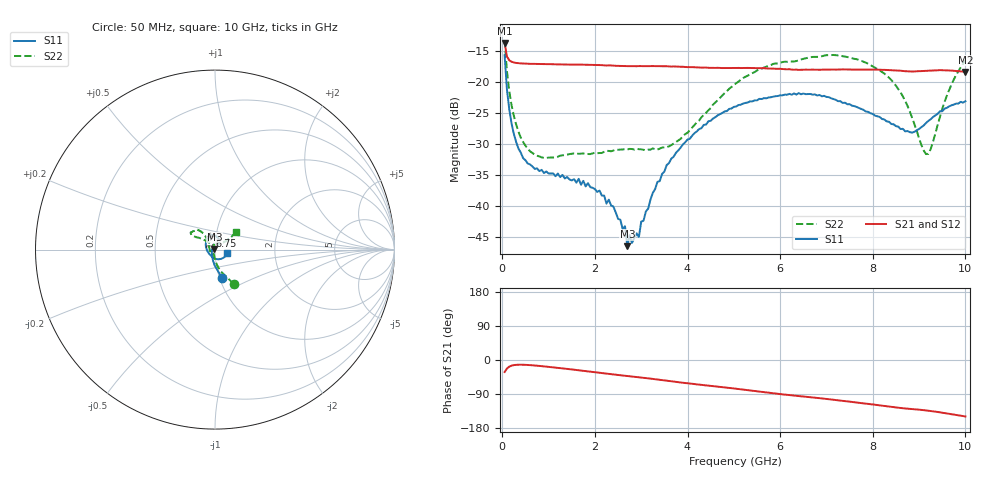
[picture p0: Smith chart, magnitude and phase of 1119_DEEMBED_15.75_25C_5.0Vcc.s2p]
!Hittite Microwave Corp.
!Digital Attenuator/PhaseShifter Rev 1.4.0
!Filename: C:\DATA\DATA\1119_DEEMBED_15.75_25C_5.0Vcc.s2p
!VNA ID: Agilent Technologies,N5224A,MY51441122,A.10.45.03
!Device type:
!2 Port Calibration.
!Temp(C): 25
!Lot Number:
!Serial Number:
!Operator:
!Misc:
!Attenuator:  15.750
# GHZ S DB R 50.0
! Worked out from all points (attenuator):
!   200 points, 50 MHz to 10 GHz, reference 50 ohm
!   highest |S21| = -13.64 dB at 50 MHz (marker M1); lowest = -18.3 dB at 10 GHz (marker M2)
!   lowest |S11| = -46.4 dB at 2.7 GHz (marker M3), VSWR 1.01, Z = 49.7 + j0.382 ohm
!   |S11| at or under -10 dB: start of sweep to end of sweep
!   |S22| runs from -32.2 to -13.2 dB; largest |S21 - S12| = 0.00047
!   S11 on the Smith chart (normalised r, x): 50 MHz: 1.03, -0.34; 6.75 GHz: 0.94, +0.14; 10 GHz: 1.14, -0.05
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0.05  -15.62 -75.7  -13.64 -31.8  -13.64 -31.8  -13.25 -61.3
0.1  -21.12 -91.5  -15.82 -22.7  -15.82 -22.7  -18.18 -75.9
0.2  -26.64 -108.2  -16.68 -14.9  -16.69 -14.9  -23.70 -87.3
0.5  -32.57 -138.9  -16.99 -12.8  -16.99 -12.7  -30.21 -99.6
0.85  -34.12 -159.5  -17.05 -16.2  -17.05 -16.2  -32.12 -106.4
1.75  -35.90 -178.8  -17.16 -28.6  -17.16 -28.6  -31.47 -116.7
2.3  -38.93 165.0  -17.27 -36.6  -17.27 -36.7  -31.07 -132.0
2.65  -43.22 131.8  -17.38 -41.6  -17.39 -41.6  -30.77 -141.7
2.7  -46.43 126.5  -17.38 -42.2  -17.39 -42.3  -30.84 -142.6
2.75  -44.64 119.1  -17.40 -42.9  -17.40 -43.0  -30.74 -144.7
2.95  -44.93 89.4  -17.38 -45.5  -17.39 -45.6  -30.79 -153.9
3.4  -35.94 62.6  -17.40 -52.2  -17.41 -52.3  -30.70 -176.9
4  -29.24 58.0  -17.55 -61.4  -17.56 -61.4  -28.14 149.1
5.05  -23.90 70.6  -17.69 -75.8  -17.71 -75.9  -20.15 125.3
6.7  -21.99 109.8  -17.96 -98.8  -17.97 -98.8  -15.91 139.8
6.75  -21.95 110.4  -17.96 -99.5  -17.97 -99.5  -15.90 140.3
7.65  -23.97 143.4  -17.94 -112.2  -17.95 -112.2  -16.27 148.3
8.35  -26.36 174.6  -18.03 -122.8  -18.03 -122.8  -19.25 143.1
8.85  -28.11 -138.6  -18.26 -129.4  -18.26 -129.4  -25.73 130.5
9.2  -26.22 -94.4  -18.12 -133.8  -18.13 -133.9  -31.54 82.9
9.6  -24.12 -54.3  -18.08 -141.1  -18.09 -141.1  -22.15 38.2
10  -23.05 -16.5  -18.33 -149.0  -18.33 -148.9  -16.47 39.8
